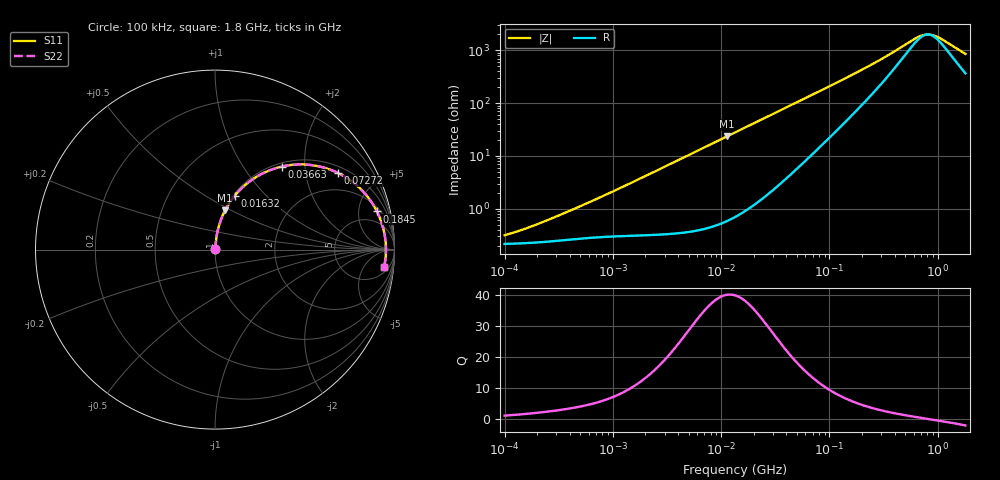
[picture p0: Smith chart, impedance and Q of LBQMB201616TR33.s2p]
! LBQMB201616TR33  S-PARAMETER MODEL  ( General Type )
! Model Generated by TAIYO YUDEN Corporation (http://www.ty-top.com)
! Version 1.0
! TAIYO YUDEN Control No. 191025NI43SB-FBB
! Copyright(c) 2019 TAIYO YUDEN CO.,LTD. All Rights Reserved.
! Product Description (link to TY-COMPAS)
! https://ds.yuden.co.jp/TYCOMPAS/or/detail?pn=LBQMB201616TR33J&u=M
! Products Name : Inductors
! Characteristics :
!  Inductance : 0.33 uH , SRF(min) : 400 MHz , DC Resistance(max) : 0.273 Ohm , Rated Current : 490 mA
!  Case Size : 2.0 x 1.6 / 0.079 x 0.063 [mm/inch] , Thickness : 1.6 / 0.063 [mm/inch]
!  (Conditions: Temperature = 25 degC , DC Bias Current/Voltage = 0A / 0V)
! External Node Assignments :
!  1  o---GGG---o  2
! GND o---------o GND
! Frequency Range : 0.1MHz  -  1800MHz  [ 402 STEP ]
# MHz S RI R 50
! Freq[MHz].  S11 Real  S11 Imag  S21 Real  S21 Imag  S12 Real  S12 Imag  S22 Real  S22 Imag
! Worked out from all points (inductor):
!   401 points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, 100 kHz to 1.8 GHz, reference 50 ohm
!   read as one part in series: L = 348 nH near 348.8 kHz
!   highest Q = 40.1 at 11.3 MHz (marker M1), where L = 330 nH
!   self-resonance near 810.1 MHz
!   S11 on the Smith chart (normalised r, x): 100 kHz: 1.00, +0.00; 16.32 MHz: 1.02, +0.68; 36.63 MHz: 1.06, +1.52; 72.72 MHz: 1.24, +3.02; 184.5 MHz: 2.57, +7.75; 1.8 GHz: 8, -15
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0.1  0.00216 0.0023  0.9978 -0.0023  0.9978 -0.0023  0.00216 0.0023
0.189057  0.0023 0.00429  0.9977 -0.00429  0.9977 -0.00429  0.0023 0.00429
0.516129  0.00285 0.0111  0.9971 -0.0111  0.9971 -0.0111  0.00285 0.0111
2.66389  0.00625 0.0549  0.9938 -0.0549  0.9938 -0.0549  0.00625 0.0549
5.833619  0.0181 0.1184  0.9819 -0.1184  0.9819 -0.1184  0.0181 0.1184
11.30236  0.057 0.2197  0.943 -0.2197  0.943 -0.2197  0.057 0.2197
13.41641  0.0773 0.2549  0.9227 -0.2549  0.9227 -0.2549  0.0773 0.2549
16.32081  0.109 0.2989  0.891 -0.2989  0.891 -0.2989  0.109 0.2989
24.15197  0.208 0.3906  0.792 -0.3906  0.792 -0.3906  0.208 0.3906
36.62703  0.3716 0.4626  0.6284 -0.4626  0.6284 -0.4626  0.3716 0.4626
50.36143  0.5217 0.4726  0.4783 -0.4726  0.4783 -0.4726  0.5217 0.4726
69.24595  0.6641 0.4365  0.3359 -0.4365  0.3359 -0.4365  0.6641 0.4365
72.72283  0.6836 0.4277  0.3164 -0.4277  0.3164 -0.4277  0.6836 0.4277
113.0207  0.8216 0.3272  0.1784 -0.3272  0.1784 -0.3272  0.8216 0.3272
184.4683  0.902 0.2129  0.098 -0.2129  0.098 -0.2129  0.902 0.2129
357.3983  0.9423 0.0975  0.0577 -0.0975  0.0577 -0.0975  0.9423 0.0975
627.8136  0.9516 0.0278  0.0484 -0.0278  0.0484 -0.0278  0.9516 0.0278
709.6131  0.9522 0.0143  0.0478 -0.0143  0.0478 -0.0143  0.9522 0.0143
802.0705  0.9524 0.00107  0.0476 -0.00107  0.0476 -0.00107  0.9524 0.00107
906.5744  0.9522 -0.0122  0.0478 0.0122  0.0478 0.0122  0.9522 -0.0122
1024.694  0.9517 -0.0256  0.0483 0.0256  0.0483 0.0256  0.9517 -0.0256
1800  0.9428 -0.0947  0.0572 0.0947  0.0572 0.0947  0.9428 -0.0947
